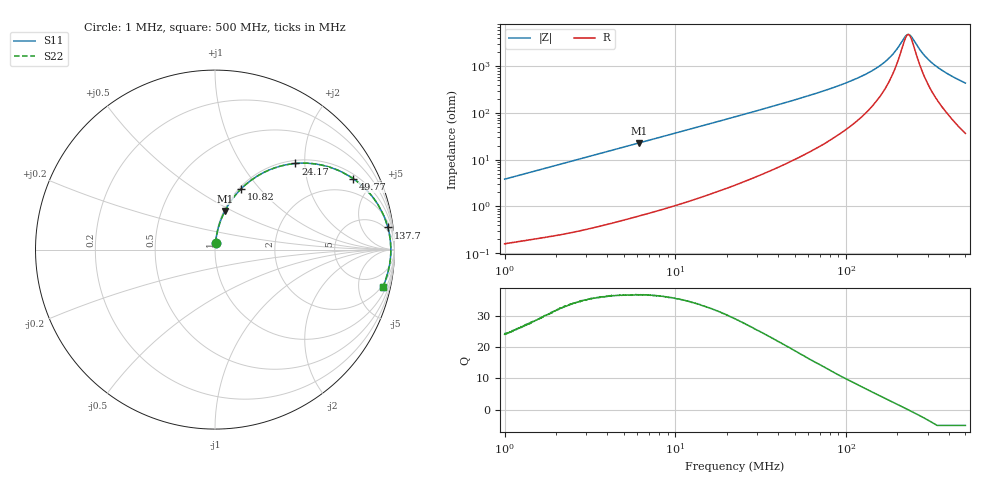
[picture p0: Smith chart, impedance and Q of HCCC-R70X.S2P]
!s-Parameter Generated by FASTRON Sdn. Bhd.
!FASTRON P/N : HCCC-R70X
!Keysight Technologies,E4991B,MY54100416,A.01.15
!Date: Thu Apr 02 13:23:32 2026
!Version  : Rev00 Thu Apr 02 13:23:32 2026
!Data & Calibration Information:
!PortZ  Port1:50+j0  Port2:50+j0
!When reading, reference impedance value at option line is always used.
!Remarks : This data is being provided solely for informational purposes.
!Freq	S11	S21	S12	S22
# Hz S dB R 50
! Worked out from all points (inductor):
!   1601 points, 1 MHz to 500 MHz, reference 50 ohm
!   read as one part in series: L = 608 nH near 1.032 MHz
!   highest Q = 36.7 at 6.134 MHz (marker M1), where L = 595 nH
!   self-resonance near 231.3 MHz
!   S11 on the Smith chart (normalised r, x): 1 MHz: 1.00, +0.08; 10.82 MHz: 1.02, +0.80; 24.17 MHz: 1.06, +1.80; 49.77 MHz: 1.20, +3.80; 137.7 MHz: 3, +15; 500 MHz: 1.73, -8.75
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1000000  -28.33 85.4  -0.02 -2.2  -0.02 -2.2  -28.33 85.4
2820919  -19.52 82.3  -0.08 -6.1  -0.08 -6.1  -19.52 82.3
6134256  -13.06 75.6  -0.27 -12.8  -0.27 -12.8  -13.06 75.6
7957584  -10.98 72.0  -0.43 -16.4  -0.43 -16.4  -10.98 72.0
1.081541e7  -8.64 66.7  -0.74 -21.7  -0.74 -21.7  -8.64 66.7
1.534122e7  -6.22 59.0  -1.33 -29.2  -1.33 -29.2  -6.22 59.0
2.236068e7  -4.04 49.1  -2.42 -38.9  -2.42 -38.9  -4.04 49.1
2.416697e7  -3.65 46.9  -2.72 -41.0  -2.72 -41.0  -3.65 46.9
3.401461e7  -2.26 37.2  -4.36 -50.4  -4.36 -50.4  -2.26 37.2
4.977112e7  -1.25 27.1  -6.83 -59.9  -6.83 -59.9  -1.25 27.1
6.307767e7  -0.84 21.5  -8.71 -64.9  -8.71 -64.9  -0.84 21.5
9.859709e7  -0.41 12.7  -13.14 -71.7  -13.14 -71.7  -0.41 12.7
1.376999e8  -0.26 7.3  -17.82 -73.3  -17.82 -73.3  -0.26 7.3
1.77937e8  -0.20 3.6  -23.58 -68.3  -23.58 -68.3  -0.20 3.6
1.96082e8  -0.19 2.3  -27.02 -60.5  -27.02 -60.5  -0.19 2.3
2.220328e8  -0.18 0.6  -32.95 -25.0  -32.95 -25.0  -0.18 0.6
2.335319e8  -0.18 -0.1  -33.78 6.4  -33.78 6.4  -0.18 -0.1
2.42781e8  -0.18 -0.7  -32.61 29.2  -32.61 29.2  -0.18 -0.7
2.835887e8  -0.19 -2.9  -25.38 65.3  -25.38 65.3  -0.19 -2.9
3.211208e8  -0.20 -4.7  -21.47 71.7  -21.47 71.7  -0.20 -4.7
3.914696e8  -0.26 -7.9  -17.15 74.0  -17.15 74.0  -0.26 -7.9
5e8  -0.37 -12.6  -13.23 72.7  -13.23 72.7  -0.37 -12.6
